(* Logix 5000 AddOnInstructionDefinition export AMP_SCL_Command_Execute; software revision 20.04 *)

TYPE AMP_Status_Word :   // Applied Motion Input Assembly Status Word
STRUCT
   Enabled : BOOL;   // Motor Enabled (Motor Disabled if this bit = 0)
   Sampling : BOOL;   // Sampling (for Quick Tuner)
   Drive_Fault : BOOL;   // Drive Fault (check Alarm Code)
   In_Position : BOOL;   // In Position (motor is in position)
   Moving : BOOL;   // Moving (motor is moving)
   Jogging : BOOL;   // Jogging (currently in jog mode)
   Stopping : BOOL;   // Stopping (in the process of stopping from a stop command)
   Waiting : BOOL;   // Waiting (for an input; executing a WI command)
   Saving : BOOL;   // Saving (parameter data is being saved)
   Alarm_Present : BOOL;   // Alarm present (check Alarm Code)
   Homing : BOOL;   // Homing (executing an SH command)
   Wait_Time : BOOL;   // Waiting (for time; executing a WD or WT command)
   Wizard_Running : BOOL;   // Wizard running (Timing Wizard is running)
   Checking_Encoder : BOOL;   // Checking encoder (Timing Wizard is running)
   Q_Program_Running : BOOL;   // Q Program is running
   Initializing : BOOL;   // Initializing (happens at power up) ; Servo Ready (for SV200 drives only)
END_STRUCT
END_TYPE

TYPE AMP_Input_Assembly_v2 :   // Applied Motion Drive Input Assembly Version 2.0
STRUCT
   Status_Code : DINT;   // Status Code
   Alarm_Code : DINT;   // Alarm Code
   Voltage : DINT;   // Supply Voltage (x0.1V)
   Current : DINT;   // Actual Current (mA)
   Temp : DINT;   // Drive Temperature (0.1 deg C)
   Encoder_Position : DINT;   // Encoder Position (20,000 counts = 1 shaft turn)
   Absolute_Position : DINT;   // Absolute Position (20,000 counts = 1 shaft turn)
   Position_Error : DINT;   // Position Error (counts)
   Actual_Velocity : DINT;   // Actual Velocity (rev/sec * 240, 0 when no encoder)
   Extended_Inputs : DINT;   // Input Status (Extended)
   Main_Board_Inputs : DINT;   // Input Status (Main board)
   Word11 : DINT;   // Reserved
   Analog_Input_1 : DINT;   // Analog Input 1 (ADC counts, 0=min V, 16383 = max V)
   Analog_Input_2 : DINT;   // Analog Input 2 (ADC counts, 0=min V, 16383 = max V)
END_STRUCT
END_TYPE

ADD_ON_INSTRUCTION AMP_SCL_Command_Execute   (* revision 1.0 *)
// Applied Motion - SCL Command Execute AOI
// Help:
// The SCL Command Execute AOI executes selected SCL commands (as listed under “Available SCL Commands” in the Host Command Reference).
VAR_IN_OUT
   Input : DINT[14]; {required}   // Drive Input Assembly
   Output : DINT[16]; {required}   // Drive Output Assembly
        [0]   // Command Word
        [1]   // Jog Speed (0.25 rev/min)
        [2]   // Jog Acceleration (10 rev/s/s)
        [3]   // Jog Deceleration (10 rev/s/s)
        [4]   // Point-to-Point Velocity (0.25 rev/min)
        [5]   // Point-to-Point Acceleration (10 rev/s/s)
        [6]   // Point-to-Point Deceleration (10 rev/s/s)
        [7]   // Point-to-Point Distance (Motor steps)
        [9]   // (2x ASCII Letters in 16 lower word)
        [10]   // Data/Register 1
        [11]   // Data/Register 2
END_VAR
VAR_INPUT
   RPI : DINT := 100; {visible}   // Drive Connection Request Packet Interval (milliseconds)
   Execute : BOOL; {required}   // Execute the SCL command
   SCL_Command : INT; {required}   // SCL Command Characters (always 2)
   Reg1 : DINT; {required}   // Data / SCL Register 1
   Reg2 : DINT; {required}   // Data / SCL Register 2
END_VAR
VAR_OUTPUT
   Sent : BOOL; {access Read Only, visible}   // Command has been sent to drive
   In_Progress : BOOL; {access Read Only, visible}   // In progress = sending command
   Done : BOOL; {access Read Only, visible}   // Command sent
   Error : BOOL; {access Read Only, visible}   // Command failed to be sent
   State : DINT := 10; {access Read Only}   // Internal state of progress
END_VAR
VAR
   Loc_StatusCode : AMP_Status_Word;
   Loc_CommandOff_Timer : TIMER;   // Timer to make sure command value was 0 before sending a new command
   Loc_CommandOn_Timer : TIMER;   // Timer to make sure command value is set long enough to be sent to drive
   Loc_Input_Assembly : AMP_Input_Assembly_v2; {access None}
   Loc_Start_ONS : BOOL; {access None}
END_VAR

ROUTINE Logic   (* ladder *)
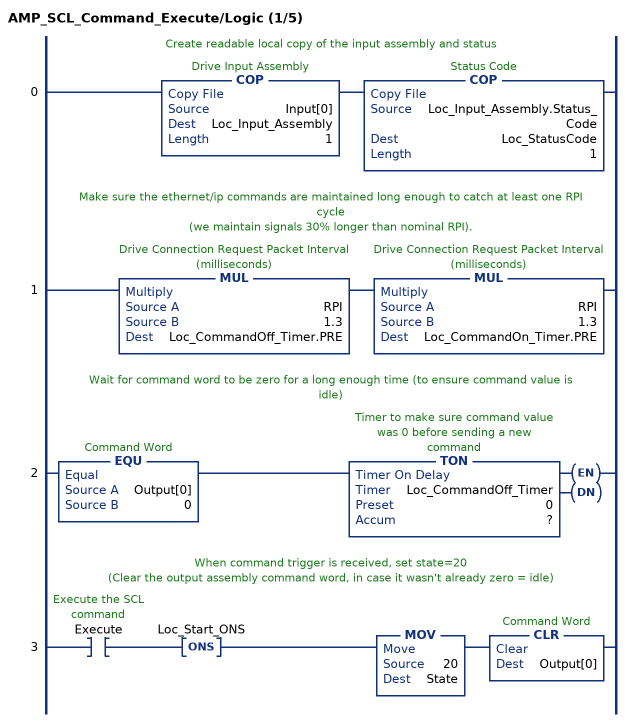
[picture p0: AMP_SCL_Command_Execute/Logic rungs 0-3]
   // Create readable local copy of the input assembly and status
   0: COP(Input[0],Loc_Input_Assembly,1)COP(Loc_Input_Assembly.Status_Code,Loc_StatusCode,1);
   // Make sure the ethernet/ip commands are maintained long enough to catch at least one RPI cycle
   // (we maintain signals 30% longer than nominal RPI).
   1: MUL(RPI,1.3,Loc_CommandOff_Timer.PRE)MUL(RPI,1.3,Loc_CommandOn_Timer.PRE);
   // Wait for command word to be zero for a long enough time (to ensure command value is idle)
   2: EQU(Output[0],0)TON(Loc_CommandOff_Timer,?,?);
   // When command trigger is received, set state=20
   // (Clear the output assembly command word, in case it wasn't already zero = idle)
   3: XIC(Execute)ONS(Loc_Start_ONS)MOV(20,State)CLR(Output[0]);
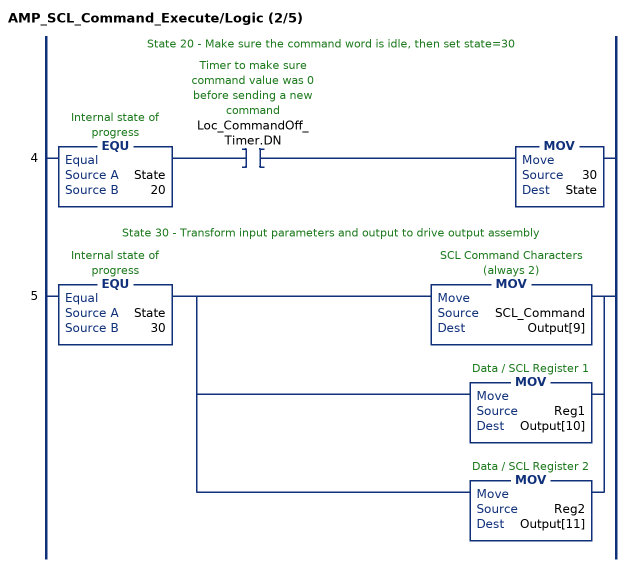
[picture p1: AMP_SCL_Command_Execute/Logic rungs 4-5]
   // State 20 - Make sure the command word is idle, then set state=30
   4: EQU(State,20)XIC(Loc_CommandOff_Timer.DN)MOV(30,State);
   // State 30 - Transform input parameters and output to drive output assembly
   5: EQU(State,30)[MOV(SCL_Command,Output[9]) ,MOV(Reg1,Output[10]) ,MOV(Reg2,Output[11]) ];
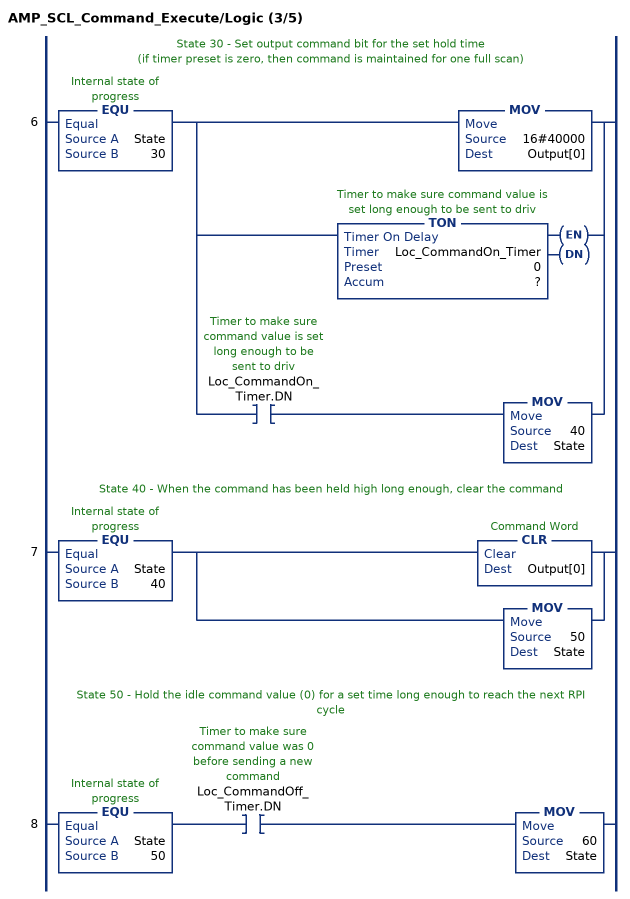
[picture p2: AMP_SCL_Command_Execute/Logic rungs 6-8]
   // State 30 - Set output command bit for the set hold time
   // (if timer preset is zero, then command is maintained for one full scan)
   6: EQU(State,30)[MOV(16#40000,Output[0]) ,TON(Loc_CommandOn_Timer,?,?) ,XIC(Loc_CommandOn_Timer.DN) MOV(40,State) ];
   // State 40 - When the command has been held high long enough, clear the command
   7: EQU(State,40)[CLR(Output[0]) ,MOV(50,State) ];
   // State 50 - Hold the idle command value (0) for a set time long enough to reach the next RPI cycle
   8: EQU(State,50)XIC(Loc_CommandOff_Timer.DN)MOV(60,State);
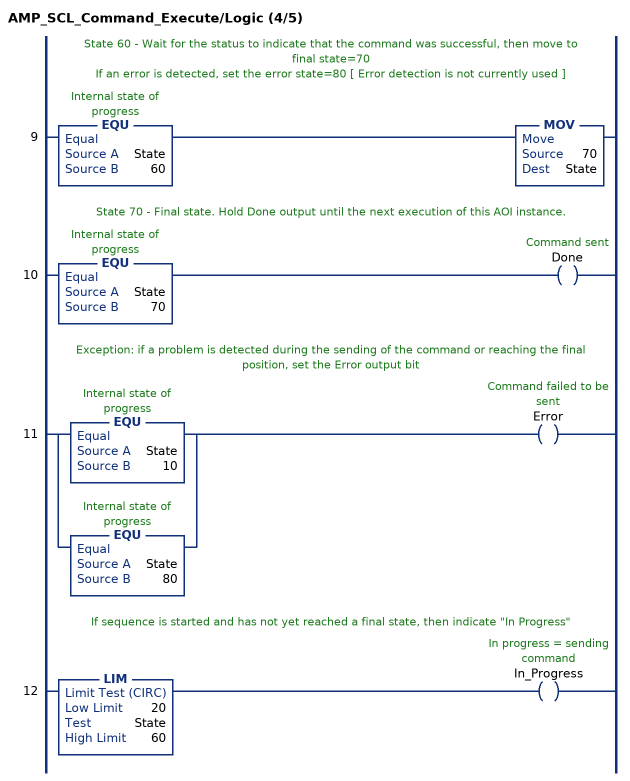
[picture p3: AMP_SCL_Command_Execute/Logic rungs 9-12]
   // State 60 - Wait for the status to indicate that the command was successful, then move to final state=70
   // If an error is detected, set the error state=80 [ Error detection is not currently used ]
   9: EQU(State,60)MOV(70,State);
   // State 70 - Final state. Hold Done output until the next execution of this AOI instance.
   10: EQU(State,70)OTE(Done);
   // Exception: if a problem is detected during the sending of the command or reaching the final position, set the Error output bit
   11: [EQU(State,10) ,EQU(State,80) ]OTE(Error);
   // If sequence is started and has not yet reached a final state, then indicate "In Progress"
   12: LIM(20,State,60)OTE(In_Progress);
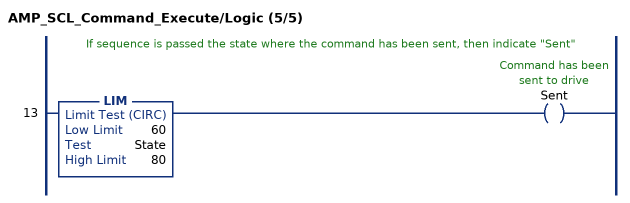
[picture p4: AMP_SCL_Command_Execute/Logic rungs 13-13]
   // If sequence is passed the state where the command has been sent, then indicate "Sent"
   13: LIM(60,State,80)OTE(Sent);
END_ROUTINE
END_ADD_ON_INSTRUCTION
